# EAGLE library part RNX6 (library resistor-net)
RESISTOR NETWORK
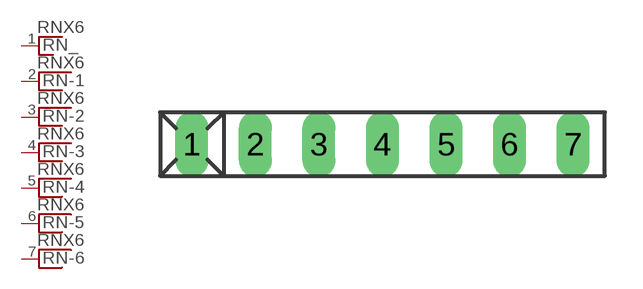
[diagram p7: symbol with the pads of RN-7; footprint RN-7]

Designator prefix RN; gates _=RN_1 -1=RNX -2=RNX -3=RNX -4=RNX -5=RNX -6=RNX

## RNX6 (OC_FARNELL: unknown; OC_NEWARK: unknown)  [RN-7]
1  _:1  pas
2  -1:1  pas
3  -2:1  pas
4  -3:1  pas
5  -4:1  pas
6  -5:1  pas
7  -6:1  pas

## Footprint RN-7 (pad centres in mm)
RESISTOR NETWORK
drill 0.813 long: 1 -7.62,0; 2 -5.08,0; 3 -2.54,0; 4 0,0; 5 2.54,0; 6 5.08,0; 7 7.62,0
